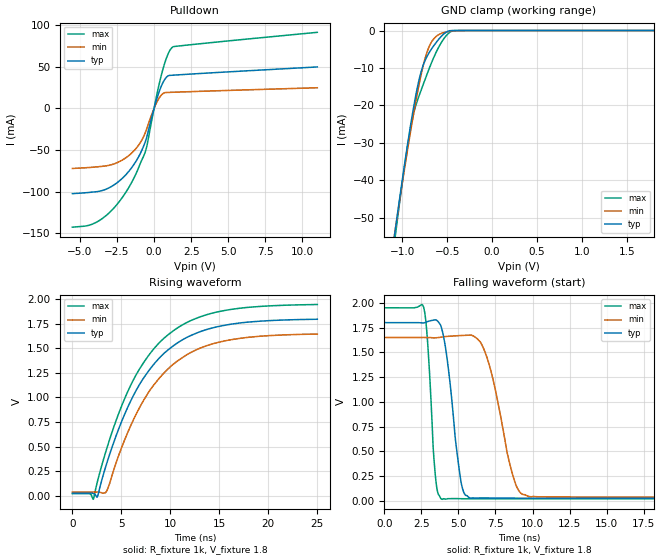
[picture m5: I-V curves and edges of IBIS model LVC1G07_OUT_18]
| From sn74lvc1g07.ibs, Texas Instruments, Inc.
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[Model]   LVC1G07_OUT_18
Model_type  Open_drain
Enable   Active-Low
Vref =   0
Rref =   1000
Cref =   30p
Vmeas =   0.9
| variable   typ   min   max
C_comp   3.53pF   2.62pF   5.10pF
| C_pulldown   8.14pF   4.54pF   12.78pF
| C_tri-state   3.53pF   2.62pF   5.10pF
[Temperature Range]   40   100   -40
| Ambient temperature   25   85   -40
[Voltage range]   1.8   1.65   1.95
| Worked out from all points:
|   slope of the pulldown table from 0 to 0.27 V, typ, clamps not added: 16.6 ohm
|   GND clamp passes 1 mA (typ) near -0.54 V on its own axis
|   rising waveform, R_fixture 1k, V_fixture 1.8: 20-80 % time 5.61ns typ, 5.58ns min, 5.63ns max; typ from 0.027 V to 1.79 V
|   falling waveform, R_fixture 1k, V_fixture 1.8: 20-80 % time 769ps typ, 1.32ns min, 421ps max; typ from 1.8 V to 0.027 V
[GND Clamp]
| LVC1G07_OUT_18
|   Voltage   I(typ)   I(min)   I(max)
-5.5V     -945.7mA   -886mA     -1.02A
-1.095V   -56.19mA   -55.94mA   -58.19mA
-1.065V   -50.97mA   -51.08mA   -52.51mA
-920mV    -27.18mA   -28.74mA   -27.7mA
-875mV    -20.66mA   -22.38mA   -22.28mA
-820mV    -13.87mA   -15.23mA   -17.9mA
-770mV    -9.464mA   -9.667mA   -14.63mA
-720mV    -6.717mA   -5.462mA   -11.4mA
-620mV    -3.107mA   -1.527mA   -5.656mA
-515mV    -495.3uA   -426.7uA   -1.484mA
-425mV    -5.264uA   -89.29uA   -16.05uA
1.8V      20.21pA    264.6pA    784.5pA
[Pulldown]
| LVC1G07_OUT_18
|   Voltage   I(typ)   I(min)   I(max)
-5.5V     -102.4mA   -72.09mA   -142.6mA
-4.355V   -100.9mA   -70.93mA   -140.2mA
-3.445V   -98.38mA   -69.44mA   -131.8mA
-2.465V   -88.93mA   -64.96mA   -114.7mA
-1.565V   -72.55mA   -54.53mA   -90.74mA
-985mV    -56.22mA   -42.66mA   -68.76mA
-570mV    -39.08mA   -28.24mA   -51mA
45mV      2.942mA    1.948mA    4.098mA
460mV     25.55mA    15.44mA    37.8mA
870mV     38.16mA    19.22mA    62.21mA
1.235V    39.96mA    19.46mA    73.59mA
11V       49.92mA    24.91mA    91.52mA
[Ramp]
| LVC1G07_OUT_18
| variable   typ   min   max
dV/dt_r   1.09/5.63E-09   0.97/5.60E-09   1.19/5.65E-09
dV/dt_f   1.08/8.30E-10   0.98/1.39E-09   1.18/4.51E-10
R_load = 1k
[Rising Waveform]
| LVC1G07_OUT_18
R_fixture =   1k
C_fixture =   0
L_fixture =   0
V_fixture =   1.8
V_fixture_min = 1.65
V_fixture_max = 1.95
|   Time   V(typ)   V(min)   V(max)
0s        26.95mV    37.1mV     21.07mV
2.135ns   23.01mV    37.18mV    -36.3mV
2.555ns   -8.156mV   37.59mV    143.9mV
3.415ns   300.9mV    35.67mV    450.1mV
4.91ns    726.6mV    460mV      884.6mV
6.435ns   1.058V     815.2mV    1.218V
8.035ns   1.303V     1.09V      1.46V
9.97ns    1.5V       1.309V     1.653V
15.27ns   1.728V     1.569V     1.879V
24.99ns   1.795V     1.644V     1.945V
[Falling Waveform]
| LVC1G07_OUT_18
R_fixture =   1k
C_fixture =   0
L_fixture =   0
V_fixture =   1.8
V_fixture_min = 1.65
V_fixture_max = 1.95
|   Time   V(typ)   V(min)   V(max)
0s        1.8V       1.65V      1.95V
2.66ns    1.797V     1.65V      1.951V
2.925ns   1.811V     1.649V     1.592V
3.435ns   1.828V     1.647V     269mV
3.865ns   1.743V     1.654V     17.28mV
5.175ns   189.6mV    1.67V      22.08mV
5.745ns   31.21mV    1.673V     21.26mV
6.93ns    29.83mV    1.446V     21.01mV
9.295ns   27.21mV    68.37mV    21.07mV
24.99ns   26.95mV    37.11mV    21.07mV
